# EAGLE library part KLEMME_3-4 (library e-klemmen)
Klemme 3 4
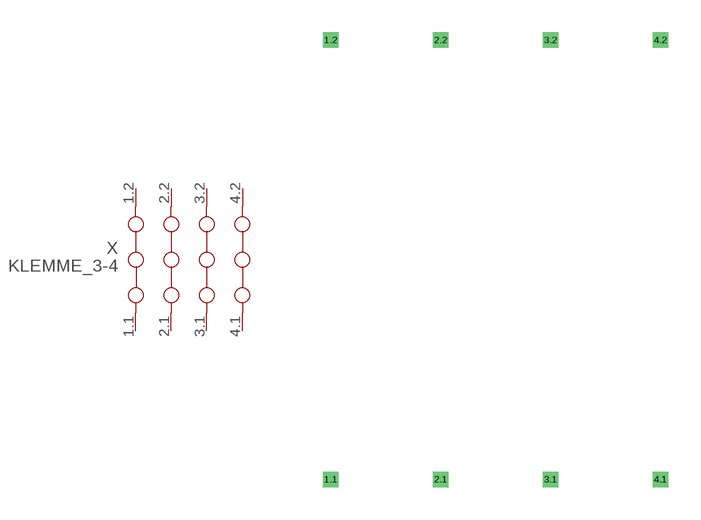
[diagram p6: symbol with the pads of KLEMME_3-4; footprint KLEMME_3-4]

Designator prefix X

## KLEMME_3-4  [KLEMME_3-4]
1.1  1.1  pas
1.2  1.2  pas
2.1  2.1  pas
2.2  2.2  pas
3.1  3.1  pas
3.2  3.2  pas
4.1  4.1  pas
4.2  4.2  pas

## Footprint KLEMME_3-4 (pad centres in mm)
Dummy
drill 0.2 pad 0.6 square: 1.1 0,-10.16; 1.2 0,10.16; 2.1 5.08,-10.16; 2.2 5.08,10.16; 3.1 10.16,-10.16; 3.2 10.16,10.16; 4.1 15.24,-10.16; 4.2 15.24,10.16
